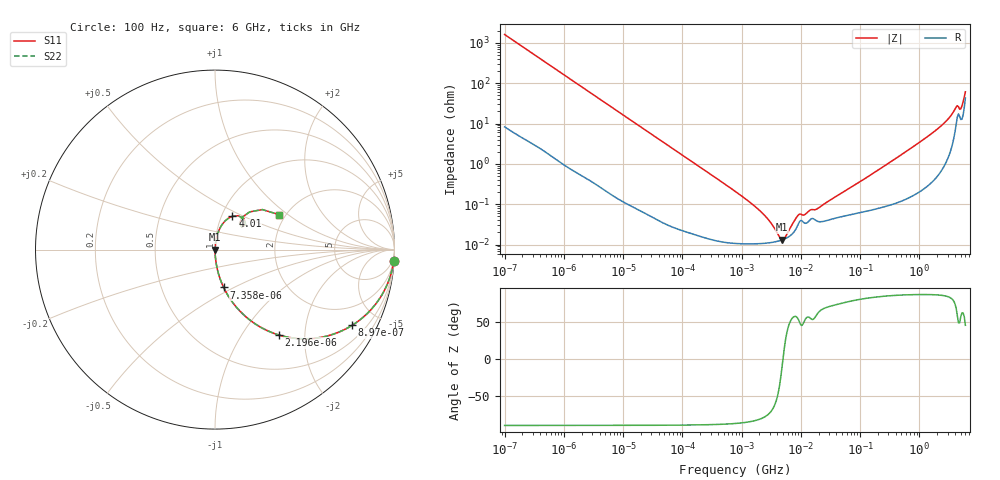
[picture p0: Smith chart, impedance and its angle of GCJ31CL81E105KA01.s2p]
!Murata Part Number: GCJ31CL81E105KA01
!These Parameters are Measured in Series Mode Connection
!Data Generated on Mar 13, 2026
!  o--ll--o
!Port1  Port2
!  o------o
!Operation Temp=25[degC], DC Bias Voltage=0[V]
!Freq. Start=100[Hz] Stop=6[GHz] 401[Steps]
# Hz S RI R 50
!Freq.(Hz) S11(Real) S11(Imag) S21(Real) S21(Imag) S12(Real) S12(Imag) S22(Real) S22(Imag)
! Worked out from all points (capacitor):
!   401 points, 100 Hz to 6 GHz, reference 50 ohm
!   read as one part in series: C = 989 nF near 109 Hz
!   lowest |Z| = 13.3 mohm at 4.857 MHz (marker M1)
!   series resonance near 5.001 MHz, so ESL is about 1 nH
!   S11 on the Smith chart (normalised r, x): 100 Hz: 1, -32; 897 Hz: 1.02, -3.61; 2.196 kHz: 1.01, -1.48; 7.358 kHz: 1.00, -0.44; 4.01 GHz: 1.13, +0.44; 6 GHz: 1.86, +0.87
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100  0.9958 -0.0619  0.00417 0.0619  0.00417 0.0619  0.9958 -0.0619
401  0.9408 -0.233  0.0592 0.233  0.0592 0.233  0.9408 -0.233
897  0.7641 -0.4216  0.2359 0.4216  0.2359 0.4216  0.7641 -0.4216
1342  0.5932 -0.4883  0.4068 0.4883  0.4068 0.4883  0.5932 -0.4883
2008  0.3963 -0.486  0.6037 0.486  0.6037 0.486  0.3963 -0.486
2196  0.3548 -0.4753  0.6452 0.4753  0.6452 0.4753  0.3548 -0.4753
3931  0.1483 -0.3521  0.8517 0.3521  0.8517 0.3521  0.1483 -0.3521
7358  0.0483 -0.211  0.9517 0.211  0.9517 0.211  0.0483 -0.211
40335  0.00205 -0.0407  0.998 0.0407  0.998 0.0407  0.00205 -0.0407
774597  0.000111 -0.0021  0.9999 0.0021  0.9999 0.0021  0.000111 -0.0021
2268635  0.000107 -0.000586  0.9999 0.000586  0.9999 0.000586  0.000107 -0.000586
4856642  0.000131 -1.98e-05  0.9999 1.98e-05  0.9999 1.98e-05  0.000131 -1.98e-05
5554849  0.000142 7.24e-05  0.9999 -7.24e-05  0.9999 -7.24e-05  0.000142 7.24e-05
9090158  0.000326 0.000434  0.9997 -0.000434  0.9997 -0.000434  0.000326 0.000434
1.555665e7  0.000445 0.00059  0.9996 -0.00059  0.9996 -0.00059  0.000445 0.00059
1.946e7  0.000376 0.000699  0.9996 -0.000699  0.9996 -0.000699  0.000376 0.000699
3.124326e8  0.00105 0.0107  0.9989 -0.0107  0.9989 -0.0107  0.00105 0.0107
1.873145e9  0.00868 0.0658  0.9913 -0.0658  0.9913 -0.0658  0.00868 0.0658
3.205649e9  0.0345 0.1316  0.9655 -0.1316  0.9655 -0.1316  0.0345 0.1316
4.009986e9  0.0974 0.1856  0.9026 -0.1856  0.9026 -0.1856  0.0974 0.1856
5.016141e9  0.1371 0.1474  0.8629 -0.1474  0.8629 -0.1474  0.1371 0.1474
6e9  0.3592 0.1941  0.6408 -0.1941  0.6408 -0.1941  0.3592 0.1941
